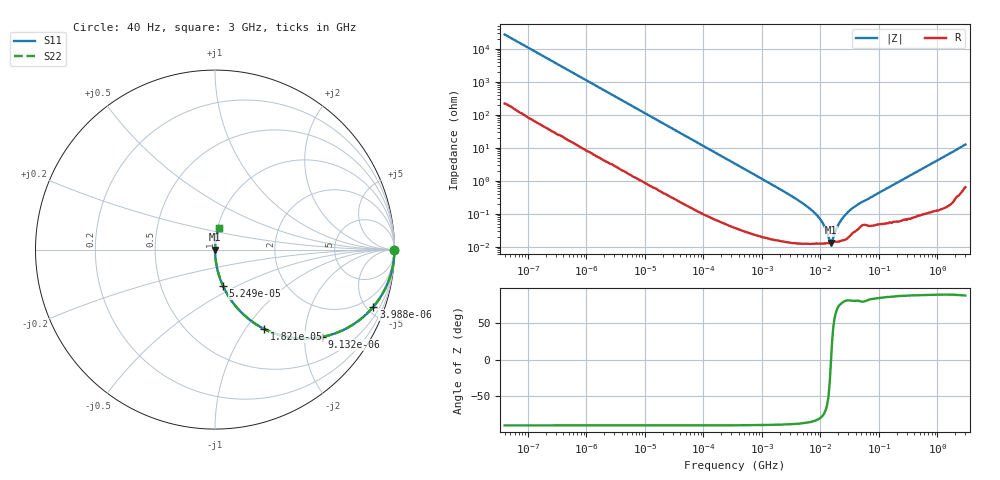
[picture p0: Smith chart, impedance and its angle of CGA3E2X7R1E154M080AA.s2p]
! S-parameter Generated by TDK Corporation
! Copyright(C) 2015 TDK Corporation.
! All Rights Reserved.
! TDK P/N: CGA3E2X7R1E154M080AA (Multilayer Ceramic Chip Capacitors)
! Property: C=150nF
! Size(LxWxT): 1.6x0.8x0.8mm, 0.063x0.031x0.031inches
! Model Type: s2p (Touchstone File Format Version 1.0)
! Frequency: DC=Yes Start=0.00004MHz Stop=3000MHz 396points Log-sweep
! Note: This model was converted from impedance.
! Model Generated on Jun. 23, 2015
! Hash(MD5):
! Port Assignments:
!  1 ---| |--- 2
! Applicable Conditions:
!  Temperature = 25 degC
!  DC Bias Voltage = 0 V
!  Small Signal Operation
! Terms and conditions regarding TDK Simulation Models
! (1)This simulation model is being provided solely for informational purposes. Please refer to the specifications of the products in terms of detailed characteristics of such products.
! (2)In no event shall TDK Corporation of any of its subsidiaries be liable for any loss or damage arising, directly or indirectly,
!  From any information contained in this simulation model, including, but not limited to loss or damages arising from any inaccuracies, omissions or errors in connection with such information.
! (3)Any and all copyrights on this simulation model are owned by TDK Corporation.
!  Duplication or redistribution of this simulation model without prior written permission from TDK Corporation is prohibited.
! (4)This simulation model is subject to any modification or change without any prior notice.
! (5)Neither TDK Corporation nor any of its subsidiaries shall make any warranty, express or implied,
!  Including but not limited to the correctness, implied warranties of merchantability and fitness for a particular purpose with respect to this simulation models.
! (6)The use of this simulation model shall be deemed to have consented to the terms and conditions hereof.
# MHz S MA R 50
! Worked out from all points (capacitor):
!   395 points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, 40 Hz to 3 GHz, reference 50 ohm
!   read as one part in series: C = 148 nF near 41.88 Hz
!   lowest |Z| = 13.2 mohm at 15.09 MHz (marker M1)
!   series resonance near 15.2 MHz, so ESL is about 740 pH
!   S11 on the Smith chart (normalised r, x): 40 Hz: open; 3.988 kHz: 1.04, -5.53; 9.132 kHz: 1.02, -2.43; 18.21 kHz: 1.01, -1.22; 52.49 kHz: 1.00, -0.43; 3 GHz: 1.01, +0.25
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4e-05  1 -0.2  0.003719 89.3  0.003719 89.3  1 -0.2
0.000834128  0.9965 -4.4  0.07593 85.2  0.07593 85.2  0.9965 -4.4
0.003988472  0.9381 -19.8  0.3393 69.7  0.3393 69.7  0.9381 -19.8
0.009132315  0.7686 -39.3  0.6338 50.2  0.6338 50.2  0.7686 -39.3
0.01739424  0.5363 -57.1  0.8398 32.4  0.8398 32.4  0.5363 -57.1
0.01821348  0.519 -58.3  0.8508 31.3  0.8508 31.3  0.519 -58.3
0.03021725  0.3451 -69.4  0.9358 20.2  0.9358 20.2  0.3451 -69.4
0.05249338  0.208 -77.5  0.9764 12.0  0.9764 12.0  0.208 -77.5
0.3464102  0.03264 -87.5  0.9991 1.9  0.9991 1.9  0.03264 -87.5
2.877491  0.003841 -87.8  0.9999 0.2  0.9999 0.2  0.003841 -87.8
7.22376  0.001235 -84.3  0.9999 0.1  0.9999 0.1  0.001235 -84.3
10.93076  0.0005194 -76.1  0.9999 0.0  0.9999 0.0  0.0005194 -76.1
12.54911  0.0003179 -66.3  0.9999 0.0  0.9999 0.0  0.0003179 -66.3
15.08561  0.0001319 -4.8  0.9999 0.0  0.9999 0.0  0.0001319 -4.8
15.79611  0.0001455 23.6  0.9999 -0.0  0.9999 -0.0  0.0001455 23.6
18.13479  0.0003056 62.4  0.9999 -0.0  0.9999 -0.0  0.0003056 62.4
20.81973  0.0005067 73.5  0.9999 -0.0  0.9999 -0.0  0.0005067 73.5
30.08671  0.001153 80.4  0.9998 -0.1  0.9998 -0.1  0.001153 80.4
47.67047  0.002106 79.2  0.9996 -0.1  0.9996 -0.1  0.002106 79.2
150.6385  0.006416 84.8  0.9994 -0.4  0.9994 -0.4  0.006416 84.8
994.0817  0.04072 85.9  0.9979 -2.3  0.9979 -2.3  0.04072 85.9
3000  0.1232 80.0  0.9861 -7.1  0.9861 -7.1  0.1232 80.0
